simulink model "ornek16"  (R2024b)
settings: Solver=VariableStepAuto  StartTime=0.0  StopTime=10.0  RelTol=1e-3
libraries: fl_lib x5, nesl_utility x2

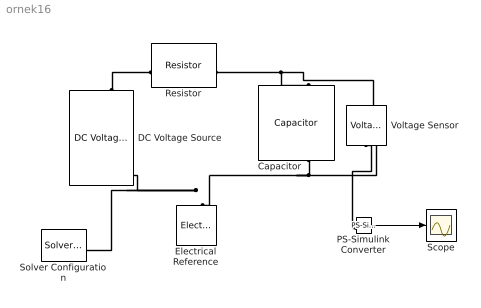
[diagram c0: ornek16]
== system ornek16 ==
  Capacitor : fl_lib/Electrical/Electrical Elements/Capacitor  c=1e-6 F  r=1e-6 Ohm  g=0 1/Ohm  i_specify=off  i_priority=None  i=0 A  i_nominal_specify=off  i_nominal_value=1  i_nominal_unit=A  v_specify=off  v_priority=None  v=0 V  v_nominal_specify=off  v_nominal_value=1  v_nominal_unit=V  vc_specify=off  vc_priority=High  vc=0 V  vc_nominal_specify=off  vc_nominal_value=1  vc_nominal_unit=V
  DC Voltage Source : fl_lib/Electrical/Electrical Sources/DC Voltage Source  v0=12 V
  Electrical Reference : fl_lib/Electrical/Electrical Elements/Electrical Reference
  PS-Simulink Converter : nesl_utility/PS-Simulink Converter  PhysicalDomain=network_engine_domain  SubClassName=ps_output  LeftPortType=input  RightPortType=output  PseudoPeriodic=off  Frequencies=[]  VectorFormat=inherit  Unit=inherit  AffineConversion=off
  Resistor : fl_lib/Electrical/Electrical Elements/Resistor  R=1 MOhm  i_specify=off  i_priority=None  i=0 A  i_nominal_specify=off  i_nominal_value=1  i_nominal_unit=A  v_specify=off  v_priority=None  v=0 V  v_nominal_specify=off  v_nominal_value=1  v_nominal_unit=V
  Scope : Scope
  Solver Configuration : nesl_utility/Solver Configuration  PhysicalDomain=network_engine_domain  SubClassName=solver  LeftPortType=input  RightPortType=generic  Tones=[]  Harmonics=[]  SimulateNoise=off  Profile=off  UseLocalSampling=off  EnableSwitchedLinearOptims=on  FrequencyDomain=off  UseCCode=off  RelTol=0.001  AbsTol=0.001  MinStep=1e-09  ToWorkspace=off  RevertToSquareIcSolve=off  NumHomotopyIterations=100  PhasorMode=off  PhasorModeNumHarmonics=1  ConsistencySolver=NEWTON_XTOL_AFTER_FTOL  IndexReductionMethod=DerivativeReplacement  DoDC=off  ResidualTolerance=1e-09  ConsistencyTolSource=GLOBAL  ConsistencyAbsTol=0.001  ConsistencyRelTol=0.001  ConsistencyTolFactor=0.001  UseLocalSolver=off  LocalSolverChoice=NE_BACKWARD_EULER_ADVANCER  ResolveIndetEquations=on  FunctionEvalNumThread=1  LocalSolverSampleTime=0.001  DoFixedCost=off  MaxNonlinIter=3  MaxModeIter=2  ComputeImpulses=off  ImpulseIterations=2  LinearAlgebra=auto  LinearAlgebraNumThread=0  EquationFormulation=NE_TIME_EF  DelaysMemoryBudget=1024  AutomaticFiltering=on  FilteringTimeConstant=0.001  PartitionStorageMethod=AS_NEEDED  PartitionMemoryBudget=1024  PartitionMethod=ROBUST  MultibodyUseLocalSolver=off  MultibodyLocalSolverChoice=ODE1  MultibodyLocalSolverSampleTime=0.001
  Voltage Sensor : fl_lib/Electrical/Electrical Sensors/Voltage Sensor
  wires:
  PS-Simulink Converter/1 -> Scope/1
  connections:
  DC Voltage Source/LConn1 -- Resistor/LConn1
  Resistor/RConn1 -- Voltage Sensor/LConn1 -- Capacitor/LConn1
  Capacitor/RConn1 -- Solver Configuration/RConn1 -- DC Voltage Source/RConn1 -- Electrical Reference/LConn1 -- Voltage Sensor/RConn2
  PS-Simulink Converter/LConn1 -- Voltage Sensor/RConn1
